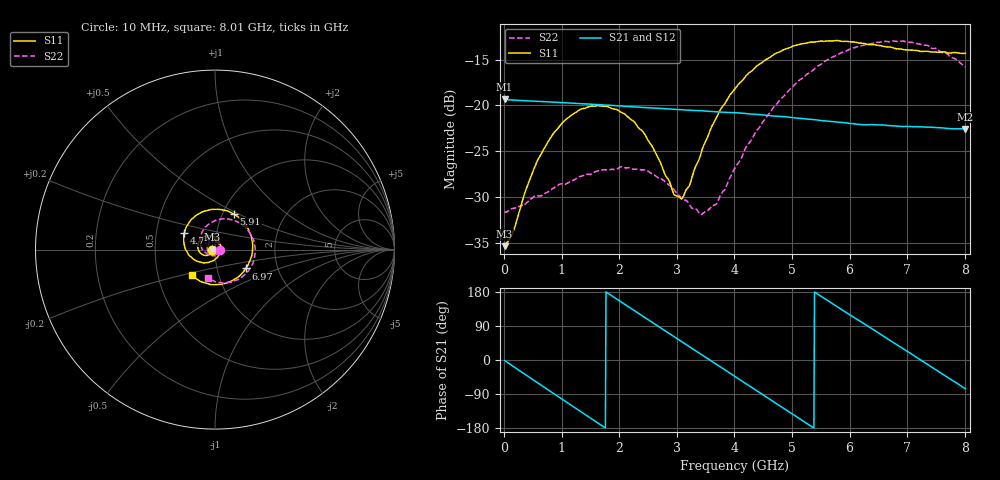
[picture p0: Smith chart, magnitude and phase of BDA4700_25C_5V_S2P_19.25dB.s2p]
!Agilent Technologies,E5071B,MY42404982,A.09.10
!Date: Mon Oct 20 13:35:59 2025
!Data & Calibration Information:
!Freq	S11:SOLT2(ON)	S21:SOLT2(ON)	S12:SOLT2(ON)	S22:SOLT2(ON)
# Hz S RI R 50
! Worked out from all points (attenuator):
!   801 points, 10 MHz to 8.01 GHz, reference 50 ohm
!   highest |S21| = -19.34 dB at 10 MHz (marker M1); lowest = -22.6 dB at 8.01 GHz (marker M2)
!   lowest |S11| = -35.4 dB at 10 MHz (marker M3), VSWR 1.03, Z = 48.3 - j0.105 ohm
!   |S11| at or under -10 dB: start of sweep to end of sweep
!   |S22| runs from -31.9 to -13.0 dB; largest |S21 - S12| = 0.00088
!   S11 on the Smith chart (normalised r, x): 10 MHz: 0.97, -0.00; 4.75 GHz: 0.70, +0.13; 5.91 GHz: 1.13, +0.47; 6.97 GHz: 1.38, -0.30; 8.01 GHz: 0.74, -0.22
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1e7  -0.017 -0.00109  0.1078 -0.00236  0.1078 -0.00245  0.0262 -0.000889
1.5e8  -0.0181 -0.00928  0.103 -0.0291  0.103 -0.0291  0.0264 -0.00722
4.1e8  -0.0272 -0.0247  0.0783 -0.0716  0.0782 -0.0717  0.0203 -0.0217
7e8  -0.0485 -0.0327  0.0323 -0.0999  0.0323 -0.0998  0.00555 -0.0325
1.02e9  -0.0776 -0.0231  -0.0261 -0.1003  -0.0261 -0.1003  -0.017 -0.0332
1.35e9  -0.0957 0.00668  -0.076 -0.0685  -0.0761 -0.0685  -0.0375 -0.0169
2.09e9  -0.0485 0.0759  -0.0836 0.0532  -0.0836 0.0533  -0.0276 0.0366
2.42e9  -0.00525 0.0713  -0.0405 0.0888  -0.0405 0.0888  -0.00168 0.0444
2.68e9  0.0212 0.0469  0.00218 0.0965  0.00218 0.0965  0.0164 0.0366
2.95e9  0.0315 0.00919  0.0449 0.0841  0.0449 0.0839  0.028 0.0206
3.09e9  0.0288 -0.0116  0.0636 0.0704  0.0633 0.0705  0.0298 0.00902
3.46e9  -0.00673 -0.0595  0.0916 0.0183  0.0917 0.0182  0.017 -0.0195
3.69e9  -0.046 -0.0726  0.0905 -0.0184  0.0905 -0.0187  -0.00166 -0.029
4.01e9  -0.1077 -0.0603  0.0664 -0.0626  0.0664 -0.0625  -0.036 -0.0277
4.75e9  -0.1713 0.0911  -0.0398 -0.0777  -0.0396 -0.0779  -0.0825 0.0623
5.35e9  -0.0631 0.2125  -0.0838 -0.00483  -0.0837 -0.00514  -0.0141 0.1537
5.91e9  0.1055 0.198  -0.0499 0.0631  -0.0501 0.063  0.1164 0.1586
6.37e9  0.1974 0.0855  0.00791 0.0783  0.00767 0.078  0.204 0.0754
6.68e9  0.208 -0.0168  0.0459 0.0628  0.0461 0.0627  0.2228 -0.00753
6.97e9  0.1716 -0.1049  0.0691 0.0337  0.0691 0.0333  0.2059 -0.0861
7.49e9  0.0279 -0.194  0.0687 -0.0321  0.0687 -0.0323  0.0959 -0.1813
8.01e9  -0.1284 -0.1439  0.0181 -0.0723  0.0182 -0.0724  -0.0388 -0.1574
